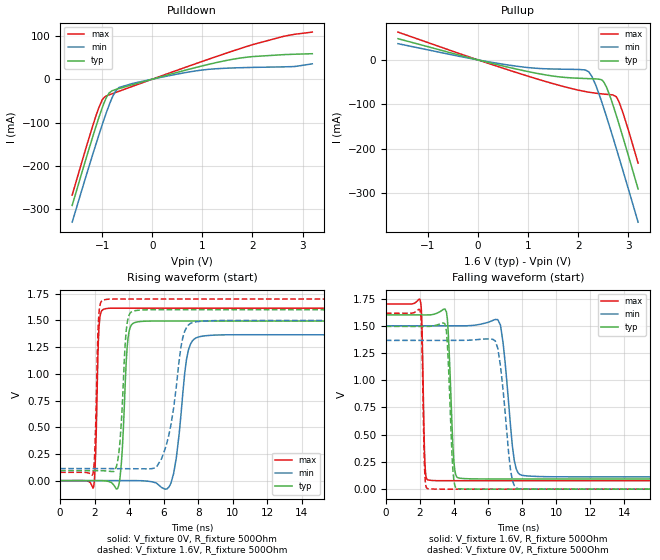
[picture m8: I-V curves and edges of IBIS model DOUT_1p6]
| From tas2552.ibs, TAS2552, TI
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|   Model
[Model]   DOUT_1p6
Model_type   Output
Polarity   Non-Inverting
Vmeas = 0.8
Vref = 0
Cref = 1pF
Rref = 1000000
|   typ   min   max
C_comp   1.241pF   1.153pF   1.378pF
[Voltage Range]   1.6   1.5   1.7
[Temperature Range]   27   125   -40
[Pullup Reference]   1.6   1.5   1.7
[Pulldown Reference]   -0   -0   -0
[Power Clamp Reference]   1.6   1.5   1.7
[GND Clamp Reference]   -0   -0   -0
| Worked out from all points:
|   slope of the pulldown table from 0 to 0.24 V, typ, clamps not added: 31.3 ohm
|   slope of the pullup table from 0 to 0.24 V, typ, clamps not added: 35.7 ohm
|   falling waveform, V_fixture 1.6V, R_fixture 500Ohm: 20-80 % time 232ps typ, 470ps min, 122ps max; typ from 1.6 V to 0.094 V
|   rising waveform, V_fixture 0V, R_fixture 500Ohm: 20-80 % time 258ps typ, 512ps min, 144ps max; typ from 0 V to 1.49 V
|   rising waveform, V_fixture 1.6V, R_fixture 500Ohm: 20-80 % time 296ps typ, 735ps min, 153ps max; typ from 0.094 V to 1.6 V
|   falling waveform, V_fixture 0V, R_fixture 500Ohm: 20-80 % time 234ps typ, 494ps min, 121ps max; typ from 1.49 V to 0 V
[Pulldown]
|   Voltage   I(typ)   I(min)   I(max)
-1.6V     -291.2mA   -329.9mA   -267.4mA
-1.187V   -132.1mA   -172.8mA   -106.9mA
-1.077V   -92.04mA   -132.4mA   -68.56mA
-1.005V   -67.66mA   -106.9mA   -48.92mA
-923.2mV  -43.92mA   -79.11mA   -39.13mA
-860.8mV  -31.85mA   -59.33mA   -36.16mA
-736mV    -24.02mA   -28.02mA   -30.87mA
-668.8mV  -21.76mA   -19.41mA   -28.04mA
675.2mV   21.14mA    15.42mA    27.9mA
1.582V    45.43mA    25.76mA    64.02mA
2.629V    56.63mA    28.42mA    99.03mA
3.195V    58.72mA    35.34mA    108.6mA
[Pullup]
|   Voltage   I(typ)   I(min)   I(max)
-1.6V     47.9mA     36.65mA    62.75mA
958.4mV   -25.35mA   -16.78mA   -35.29mA
1.597V    -37.89mA   -20.72mA   -56.63mA
2.139V    -41.94mA   -22.61mA   -71.25mA
2.206V    -42.22mA   -26.59mA   -72.61mA
2.274V    -42.48mA   -37.4mA    -73.82mA
2.35V     -42.79mA   -57.05mA   -75.03mA
2.504V    -48.86mA   -106.8mA   -76.96mA
2.571V    -63.05mA   -130.4mA   -77.65mA
2.768V    -128mA     -202.7mA   -84.44mA
2.893V    -174.4mA   -249.7mA   -119.1mA
3.195V    -291.1mA   -365.9mA   -232.7mA
[Ramp]
R_load = 500
|   typ   min   max
dV/dt_r   0.896442/2.58487e-10   0.819506/5.11747e-10   0.968975/1.43984e-10
dV/dt_f   0.903756/2.3181e-10   0.83214/4.70242e-10   0.973375/1.22293e-10
[Falling Waveform]
V_fixture = 1.6V
V_fixture_min = 1.5V
V_fixture_max = 1.7V
R_fixture = 500Ohm
C_fixture = 0F
|   Time   V(typ)   V(min)   V(max)
0s        1.6V       1.5V       1.7V
2.011ns   1.6V       1.5V       1.737V
2.314ns   1.599V     1.5V       179.6mV
2.635ns   1.601V     1.5V       80.86mV
3.556ns   1.627V     1.5V       77.72mV
3.989ns   264.5mV    1.499V     77.68mV
4.361ns   100.5mV    1.499V     77.68mV
6.736ns   93.7mV     1.506V     77.68mV
8.305ns   93.7mV     121.5mV    77.68mV
100ns     93.74mV    113.1mV    77.71mV
[Rising Waveform]
V_fixture = 0V
V_fixture_min = 0V
V_fixture_max = 0V
R_fixture = 500Ohm
C_fixture = 0F
|   Time   V(typ)   V(min)   V(max)
0s        962.6pV    31.74nV    348.3pV
1.941ns   209.1uV    158.2uV    -58.11mV
2.265ns   243.9uV    184.6uV    1.462V
2.749ns   -5.636mV   224.1uV    1.613V
3.398ns   -45.21mV   276.9uV    1.615V
4.652ns   1.49V      -606.6uV   1.615V
6.426ns   1.494V     -22.38mV   1.615V
7.438ns   1.494V     1.224V     1.615V
8.561ns   1.494V     1.359V     1.615V
100ns     1.494V     1.366V     1.615V
[Rising Waveform]
V_fixture = 1.6V
V_fixture_min = 1.5V
V_fixture_max = 1.7V
R_fixture = 500Ohm
C_fixture = 0F
|   Time   V(typ)   V(min)   V(max)
0s        93.74mV    113.1mV    77.71mV
1.906ns   93.37mV    113.1mV    65.26mV
2.241ns   93.11mV    113mV      1.549V
2.749ns   89.41mV    112.7mV    1.698V
3.327ns   176.3mV    112.2mV    1.7V
4.478ns   1.595V     111.1mV    1.7V
5.88ns    1.6V       205.7mV    1.7V
7.11ns    1.6V       1.34V      1.7V
8.124ns   1.6V       1.492V     1.7V
100ns     1.6V       1.5V       1.7V
[Falling Waveform]
|Gnd
V_fixture = 0V
V_fixture_min = 0V
V_fixture_max = 0V
R_fixture = 500Ohm
C_fixture = 0F
|   Time   V(typ)   V(min)   V(max)
0s        1.494V     1.366V     1.615V
2.011ns   1.494V     1.366V     1.638V
2.289ns   1.494V     1.366V     127.4mV
2.489ns   1.494V     1.366V     3.558mV
3.556ns   1.451V     1.366V     -11.56uV
3.935ns   178.2mV    1.366V     -11.52uV
4.206ns   4.302mV    1.366V     -11.48uV
6.426ns   -17.54uV   1.362V     -11.22uV
7.876ns   -17.26uV   2.917mV    -11.04uV
100ns     993.4pV    31.77nV    347.7pV
